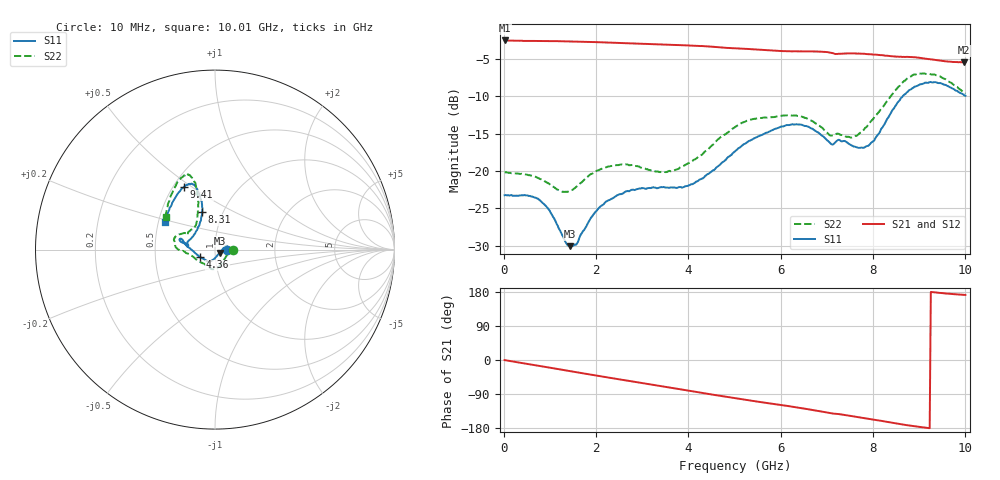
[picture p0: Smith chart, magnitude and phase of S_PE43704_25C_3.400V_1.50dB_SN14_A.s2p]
! Device ID: PE43704
! Dir: z:\PE43704\PE43704_Char_1_20130516\PE43704\AMB\3p400V\1p50dB
! Serial: 14
! Insertion: A
! Impedance: 50 ohm
! Temp: Amb
! VDD: 3.400V
! Attenuation Step: 1.50dB
! IDD: 1.141170e-01mA
#  Hz  S  RI  R  50
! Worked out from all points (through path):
!   401 points, 10 MHz to 10.01 GHz, reference 50 ohm
!   highest |S21| = -2.52 dB at 10 MHz (marker M1); lowest = -5.5 dB at 9.985 GHz (marker M2)
!   group delay of S21, straight-line fit = 53.5 ps
!   lowest |S11| = -30.1 dB at 1.435 GHz (marker M3), VSWR 1.06, Z = 52.6 - j1.93 ohm
!   |S11| at or under -10 dB: start of sweep to 8.649 GHz
!   |S22| runs from -22.8 to -6.9 dB; largest |S21 - S12| = 0.0054
!   S11 on the Smith chart (normalised r, x): 10 MHz: 1.15, +0.00; 4.36 GHz: 0.84, -0.07; 8.31 GHz: 0.80, +0.35; 9.41 GHz: 0.57, +0.47; 10.01 GHz: 0.54, +0.19
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1e7  0.0688 0.000269  0.7479 -0.00297  0.748 -0.00281  0.0981 3.09e-05
7.6e8  0.0607 0.0211  0.7142 -0.1995  0.7142 -0.1995  0.089 0.00506
9.85e8  0.0526 0.0142  0.6954 -0.2553  0.6952 -0.255  0.0814 -0.00787
1.435e9  0.0255 -0.0183  0.6417 -0.3624  0.6414 -0.3624  0.0542 -0.0497
1.685e9  0.00978 -0.0371  0.6042 -0.417  0.6043 -0.417  0.038 -0.075
2.235e9  -0.0164 -0.0607  0.5055 -0.5191  0.5059 -0.5188  0.00555 -0.1062
2.735e9  -0.0305 -0.0673  0.403 -0.5911  0.403 -0.591  -0.0203 -0.1075
3.36e9  -0.0353 -0.0687  0.2632 -0.6534  0.2639 -0.653  -0.039 -0.0907
3.91e9  -0.054 -0.0568  0.1323 -0.6815  0.133 -0.6816  -0.0853 -0.0675
4.36e9  -0.0824 -0.0416  0.0229 -0.6833  0.0237 -0.6841  -0.1307 -0.0345
5.01e9  -0.1352 0.00267  -0.1218 -0.6515  -0.1213 -0.6517  -0.1967 -0.00326
6.035e9  -0.1897 0.0598  -0.3099 -0.554  -0.3078 -0.5551  -0.2288 0.0517
6.685e9  -0.1875 0.0421  -0.4209 -0.4708  -0.4213 -0.47  -0.1988 0.0845
7.085e9  -0.1501 0.0273  -0.4754 -0.3974  -0.4774 -0.3978  -0.1502 0.0854
7.585e9  -0.131 0.0639  -0.5246 -0.3169  -0.5237 -0.3166  -0.1104 0.1292
7.935e9  -0.0973 0.115  -0.552 -0.248  -0.5531 -0.2498  -0.0984 0.1858
8.31e9  -0.0714 0.2109  -0.5659 -0.1718  -0.5639 -0.1743  -0.0956 0.2776
8.36e9  -0.0703 0.2237  -0.5658 -0.1601  -0.5655 -0.1632  -0.0945 0.2923
8.835e9  -0.1008 0.3381  -0.5756 -0.063  -0.5715 -0.0645  -0.1363 0.4087
9.41e9  -0.1726 0.3482  -0.5505 0.0233  -0.5503 0.0242  -0.199 0.3853
9.985e9  -0.2745 0.1661  -0.5284 0.0748  -0.5308 0.0763  -0.2726 0.1897
1.001e10  -0.2791 0.1541  -0.53 0.0764  -0.5333 0.0772  -0.2754 0.1802
